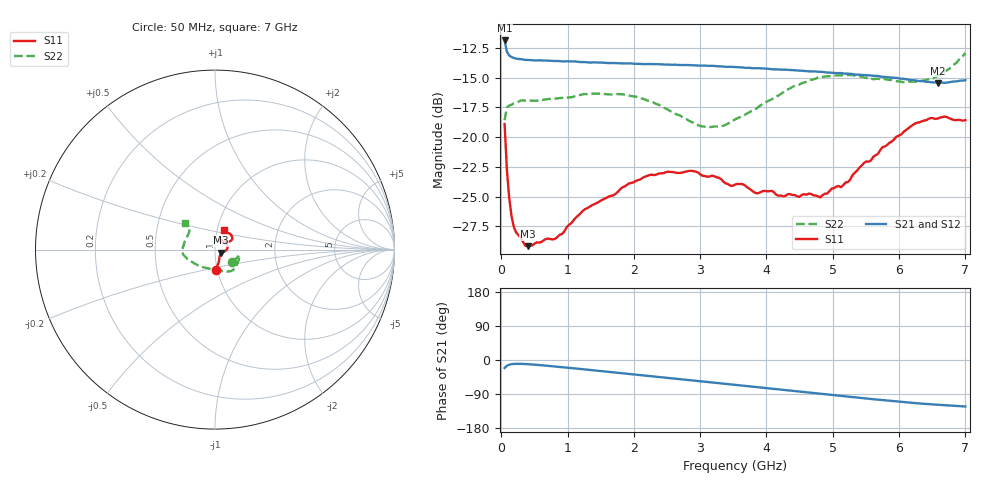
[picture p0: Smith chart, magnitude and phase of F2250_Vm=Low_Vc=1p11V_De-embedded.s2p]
! Integrated Device Technology
! Corporate Headquarters
! 6024 Silver Creek Valley Road
! San Jose, CA 95138  USA
! Phone:  1-408-284-8200
! Toll Free:  1-800-223-1366
! Webpage:  http://www.idt.com/
! Timing and RF Division
! 515 Groton Road, Suite 102
! Westford, MA 01886-6024
! Device:  F2250
! Description: Voltage Variable RF Attenuator
! Frequency:  50.0 -  6000.00 MHz
! Package:  3x3 mm Thin QFN Plastic Package: 16 pin
! Ports:  2 RF, 3 DC
!  Pin  1  = GND
!  Pin  2  = NC
!  Pin  3  = RF1  = Port 1
!  Pin  4  = NC
!  Pin  5  = GND
!  Pin  6  = GND
!  Pin  7  = GND
!  Pin  8  = GND
!  Pin  9  = NC
!  Pin 10  = RF2  = Port 2
!  Pin 11  = NC
!  Pin 12  = GND
!  Pin 13  = GND
!  Pin 14  = VCNTRL
!  Pin 15  = VDD
!  Pin 16  = VMODE
! Vcntrl:  1.110 Volts
! Vmode:  +0.000 Volts
! Vdd:  +3.30  Volts
! Current:  1.191 mA
! Data:  The device was measured on a the F2250 evaluation board which has
!  individual transmission lines to the RF pins.  Data was collected
!  using a calibrated network analyzer.  The evaluation board was
!  de-embedded using a TRL calibration technique.
!  The reference plane is the edge of the package pin.
! Misc:  SN 10
!  Action Tracker AT0258
! Date Measured:  2014-11-26
! Date:  2015-10-15  MJV
! Note:
!  Integrated Device Technology supplies this data as a sample of measured
!  data at the package pin for this product.  Your particular data for this
!  product may vary.
!  Data was taken at 25 degrees C.
!  Integrated Device Technology reserves the right to change this data at anytime.
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# GHz S dB R 50
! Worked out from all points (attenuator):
!   201 points, 50 MHz to 7 GHz, reference 50 ohm
!   highest |S21| = -11.87 dB at 50 MHz (marker M1); lowest = -15.4 dB at 6.583 GHz (marker M2)
!   lowest |S11| = -29.2 dB at 397.5 MHz (marker M3), VSWR 1.07, Z = 53.1 - j1.73 ohm
!   |S11| at or under -10 dB: start of sweep to end of sweep
!   |S22| runs from -19.1 to -12.9 dB; largest |S21 - S12| = 0.00073
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0.05  -18.89 -88.2  -11.87 -21.0  -11.87 -21.0  -18.57 -34.3
0.08475  -22.76 -73.0  -12.82 -15.2  -12.82 -15.2  -17.50 -18.5
0.1195  -25.11 -64.3  -13.14 -12.4  -13.13 -12.4  -17.35 -14.1
0.15425  -26.64 -57.0  -13.26 -11.0  -13.26 -11.0  -17.27 -12.8
0.22375  -28.00 -43.0  -13.40 -10.1  -13.39 -10.0  -17.10 -12.9
0.3975  -29.16 -27.9  -13.51 -11.0  -13.49 -11.0  -16.92 -15.0
0.8145  -28.54 -17.4  -13.60 -17.2  -13.60 -17.2  -16.76 -27.4
1.2315  -26.18 -15.0  -13.69 -24.3  -13.69 -24.3  -16.39 -38.4
1.857  -24.14 -3.4  -13.81 -35.3  -13.79 -35.3  -16.41 -51.1
2.37825  -23.05 8.5  -13.87 -44.6  -13.88 -44.6  -17.27 -63.2
2.86475  -22.82 23.4  -13.96 -53.5  -13.96 -53.5  -18.70 -83.1
3.0385  -23.24 29.4  -13.98 -56.7  -13.98 -56.7  -19.10 -93.0
3.3165  -23.53 39.9  -14.05 -61.8  -14.05 -61.9  -19.08 -111.2
3.525  -23.98 46.0  -14.12 -65.7  -14.12 -65.7  -18.51 -124.0
3.83775  -24.70 57.4  -14.21 -71.4  -14.20 -71.4  -17.63 -140.3
4.7065  -24.89 60.7  -14.47 -87.3  -14.47 -87.3  -15.15 -168.9
4.81075  -25.06 56.5  -14.50 -89.2  -14.49 -89.2  -14.93 -170.8
5.1235  -24.21 46.6  -14.61 -94.9  -14.63 -94.9  -14.81 -177.8
5.85325  -20.48 29.2  -14.98 -107.6  -14.99 -107.6  -15.19 165.1
6.2355  -18.87 31.6  -15.22 -113.7  -15.22 -113.8  -15.34 152.3
6.583  -18.43 41.2  -15.44 -118.0  -15.43 -118.0  -14.81 141.6
7  -18.57 65.9  -15.21 -122.7  -15.21 -122.8  -12.92 138.7
